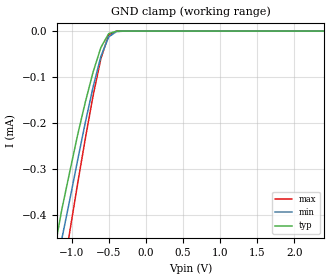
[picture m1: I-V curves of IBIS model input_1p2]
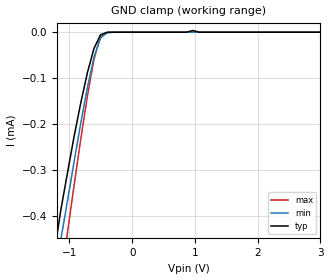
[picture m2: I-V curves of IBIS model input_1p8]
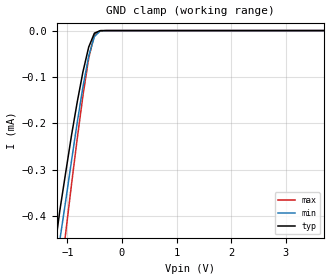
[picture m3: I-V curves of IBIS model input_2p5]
| Texas Instruments Incorporated
| SN74LXC1T14 Single-Channel Dual Supply Inverting Voltage Translator
| with Schmitt-trigger Inputs
[IBIS Ver]   4.1
[File name]   sn74lxc1t14.ibs
[File Rev]   1.0
[Date]   04/24/2019
[Source]
| Texas Instruments Incorporated.
| Analog-eLab Design Center, HPA
| 12500 TI Blvd
| Dallas, TX -75243
[Notes]   Revision History:
| Rev 1.0: 04/14/2022
| - Initial version of the model
| - Model generated from simulations in SPECTRE
| - C_comp although listed in numerical order of value are
|   obtained from varying PVT conditions. For PVT conditions for
|   each specific value refer the buffer description under
|   respective [Model]. IBIS model user is responsible for using
|   appropriate C_comp to simulate for Signal Integrity.
| - Warnings regarding combined Non-monotonicity of various models have been
|   reviewd and considered minor and can be ignored.
| - Model names with a trailing _2p5 contain the model for 2.5V operation.
[Disclaimer]
| This model is designed as an aid for customers of Texas Instruments.
| TI and its licensors and suppliers make no warranties, either expressed
| or implied, with respect to this  model, including the warranties of
| merchantability or fitness for a particular purpose. The model is
| provided solely on an "as is" basis. The entire risk as to its quality
| and performance is with the customer.
| This model is subject to change without notice. Texas Instruments
| Incorporated is not responsible for updating this model.
[Copyright]
 (C) Copyright 2022 Texas Instruments Incorporated.All rights reserved.
|Component SN74LXC1T14DCK 5-pin SOT - DCK package
|  Part # SN74LXC1T14DCK
[Component]   SN74LXC1T14DCK
[Manufacturer]  TI
[Package]   |5 SOT - DCK package
|   typ   min   max
R_pkg   0.05   0.04   0.06
L_pkg   1.0nH   0.8nH   1.2nH
C_pkg   0.2pF   0.16pF   0.24pF
[Pin]  signal_name model_name   R_pin   L_pin   C_pin
1   VCCI   power   NA   NA   NA
2   A   input   NA   NA   NA
3   GND   gnd   NA   NA   NA
4   Y   output   NA   NA   NA
5   VCCO   power   NA   NA   NA
|   Model Selectors
[Model Selector] input
input_1p2   1.2V   digital input
input_1p8   1.8V   digital input
input_2p5   2.5V   digital input
input_3p3   3.3V   digital input
input_5p0   5.0V   digital input
[Model Selector] output
output_1p2   1.2V   Vcc
output_1p8   1.8V   Vcc
output_2p5   2.5V   Vcc
output_3p3   3.3V   Vcc
output_5p0   5.0V   Vcc
| Models and submodels in the file (10): input_1p2 (Input), input_1p8 (Input), input_2p5 (Input), input_3p3 (Input), input_5p0 (Input), output_1p2 (Output), output_1p8 (Output), output_2p5 (Output), output_3p3 (Output), output_5p0 (Output)
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|   input_1p2 Model
[Model]   input_1p2
Model_type   Input
Vinl = 0.2
Vinh = 0.9
|   typ   min   max
C_comp   0.119pF   0.105pF   0.126pF
[Voltage Range]   1.2   1.08   1.32
|Junction Temperature
[Temperature Range]   25   125   -40
[GND Clamp Reference]   0   0   0
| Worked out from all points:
|   GND clamp passes 1 mA (typ) near -1.81 V on its own axis
[GND Clamp]
|   Voltage   I(typ)   I(min)   I(max)
-2.5V     -1.66mA    -1.64mA    -2.09mA
-1.24V    -478uA     -541uA     -650uA
-1.14V    -389uA     -453uA     -542uA
-1.03V    -305uA     -366uA     -435uA
-925mV    -226uA     -281uA     -332uA
-820mV    -154uA     -198uA     -233uA
-715mV    -88.7uA    -121uA     -140uA
-610mV    -35.6uA    -54.9uA    -59.7uA
-505mV    -5.5uA     -12.7uA    -8.49uA
-400mV    -210nA     -1.13uA    -141nA
8V        3.62nA     3.43nA     4.23nA
|   input_1p8 Model
[Model]   input_1p8
Model_type   Input
Vinl = 0.7
Vinh = 1.1
|   typ   min   max
C_comp   3.13pF   2.65pF   3.82pF
| Where Nom  PVT is Nominal Process, 2.25V, 27C
|   Fast PVT is Strong Process,  2.50V, -55C
|   Slow PVT is Weak Process,   2.0V, 150C
[Voltage Range]   1.8   1.62   1.98
|Junction Temperature
[Temperature Range]   25   125   -40
[GND Clamp Reference]   0   0   0
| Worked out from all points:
|   GND clamp passes 1 mA (typ) near -1.81 V on its own axis
[GND Clamp]
|   Voltage   I(typ)   I(min)   I(max)
-2.5V     -1.66mA    -1.64mA    -2.09mA
-1.24V    -478uA     -541uA     -650uA
-1.14V    -389uA     -453uA     -542uA
-1.03V    -305uA     -366uA     -435uA
-820mV    -154uA     -198uA     -233uA
-715mV    -88.7uA    -121uA     -140uA
-610mV    -35.6uA    -54.9uA    -59.7uA
-505mV    -5.5uA     -12.7uA    -8.49uA
-400mV    -210nA     -1.13uA    -141nA
965mV     3.74uA     3.02nA     4.93nA
1.07V     3.25nA     2.95nA     3.92nA
8V        3.62nA     3.43nA     4.23nA
|   input_2p5 Model
[Model]   input_2p5
Model_type   Input
Vinl = 1.0
Vinh = 1.4
|   typ   min   max
C_comp   3.03pF   2.54pF   3.83pF
| Where Nom  PVT is Nominal Process, 2.25V, 27C
|   Fast PVT is Strong Process,  2.50V, -55C
|   Slow PVT is Weak Process,   2.0V, 150C
[Voltage Range]   2.5   2.25   2.75
|Junction Temperature
[Temperature Range]   25   125   -40
[GND Clamp Reference]   0   0   0
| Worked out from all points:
|   GND clamp passes 1 mA (typ) near -1.81 V on its own axis
[GND Clamp]
|   Voltage   I(typ)   I(min)   I(max)
-2.5V     -1.66mA    -1.64mA    -2.09mA
-1.24V    -478uA     -541uA     -650uA
-1.14V    -389uA     -453uA     -542uA
-1.03V    -305uA     -366uA     -435uA
-925mV    -226uA     -281uA     -332uA
-820mV    -154uA     -198uA     -233uA
-715mV    -88.7uA    -121uA     -140uA
-610mV    -35.6uA    -54.9uA    -59.7uA
-505mV    -5.5uA     -12.7uA    -8.49uA
-400mV    -210nA     -1.14uA    -141nA
8V        3.62nA     3.43nA     4.23nA
